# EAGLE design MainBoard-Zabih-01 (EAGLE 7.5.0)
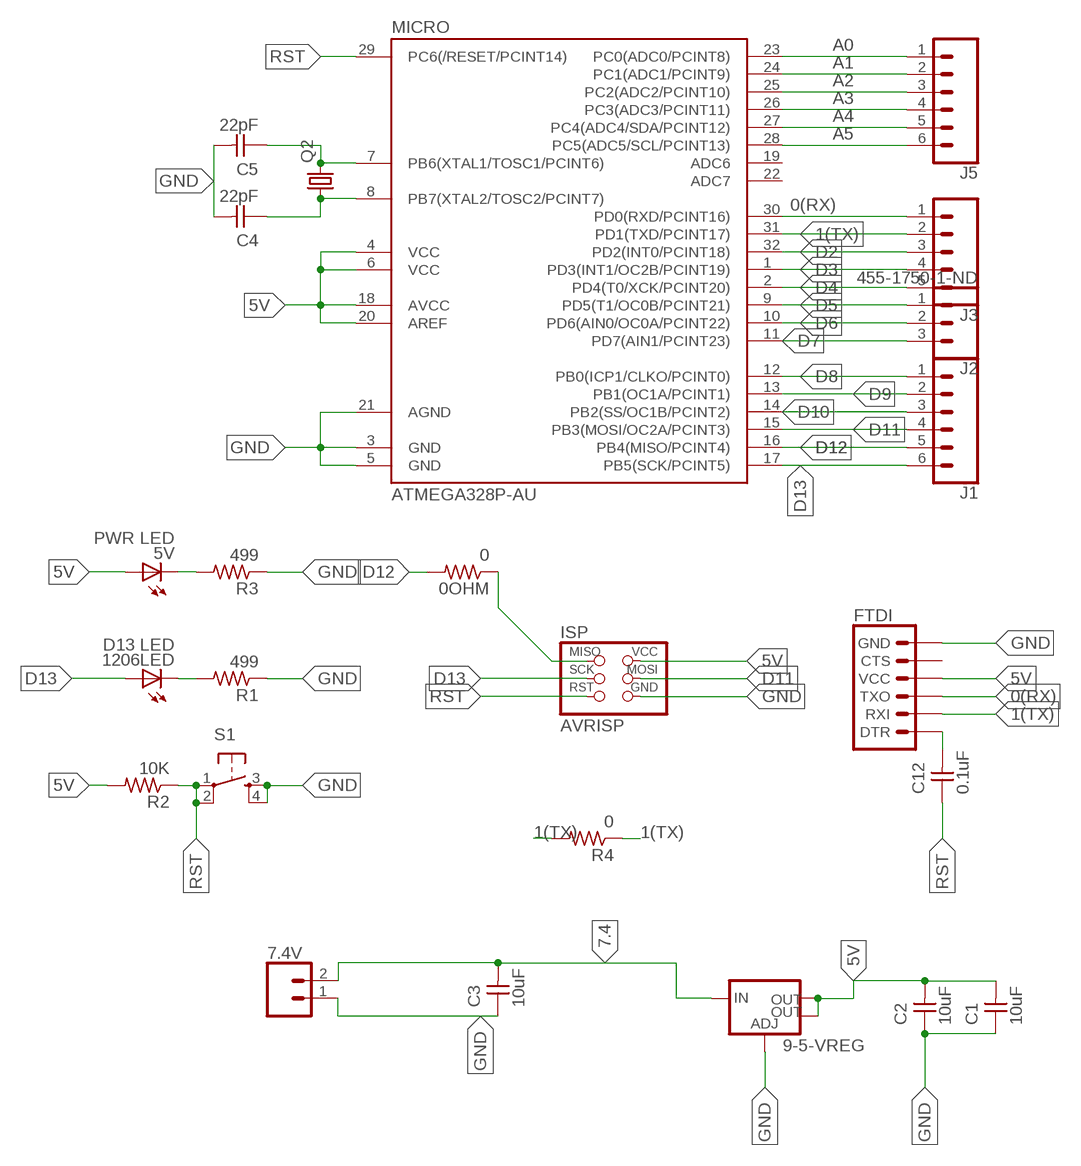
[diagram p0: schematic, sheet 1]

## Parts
0OHM  0  RES-US1206FAB  [R1206FAB]
5V  PWR LED  LEDFAB1206  [LED1206FAB]
7.4V  CONN_02LOCK  [1X02_LOCK]
9-5-VREG  V_REG_LM1117SOT223  [SOT223]
1206LED  D13 LED  LEDFAB1206  [LED1206FAB]
C1  10uF  CAP-UNPOLARIZEDFAB  [C1206FAB]
C2  10uF  CAP-UNPOLARIZEDFAB  [C1206FAB]
C3  10uF  CAP-UNPOLARIZEDFAB  [C1206FAB]
C4  22pF  CAP-UNPOLARIZEDFAB  [C1206FAB]
C5  22pF  CAP-UNPOLARIZEDFAB  [C1206FAB]
C12  0.1uF  CAP-UNPOLARIZEDFAB  [C1206FAB]
FTDI  6_PIN_SERIAL_TARGET_SILK  [1X06]
ISP  AVRISP  [2X03]
J1  CONN_06SILK_FEMALE_PTH  [1X06]
J2  455-1750-1-ND  CONN_03  [1X03]
J3  CONN_05  [1X05]
J5  CONN_06SILK_FEMALE_PTH  [1X06]
MICRO  ATMEGA328P-AU  ATMEGA48/88/168-AU  [TQFP32-08]
Q2  CRYSTALHC49U70  [HC49U70]
R1  499  RES-US1206FAB  [R1206FAB]
R2  10K  RES-US1206FAB  [R1206FAB]
R3  499  RES-US1206FAB  [R1206FAB]
R4  0  RES-US1206FAB  [R1206FAB]
S1  6MM_SWITCH6MM_SWITCH  [6MM_SWITCH]

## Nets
0(RX): FTDI.3(TXO) J3.1 MICRO.30(PD0(RXD/PCINT16))
1(TX): FTDI.2(RXI) J3.2 MICRO.31(PD1(TXD/PCINT17)) R4.1 R4.2
5V: 5V.1(A) 9-5-VREG.2(OUT) 9-5-VREG.4(OUT) C1.2 C2.2 FTDI.4(VCC) ISP.2(VCC) MICRO.4(VCC) MICRO.6(VCC) MICRO.18(AVCC) MICRO.20(AREF) R2.2
7.4: 7.4V.2 9-5-VREG.3(IN) C3.2
A0: J5.1 MICRO.23(PC0(ADC0/PCINT8))
A1: J5.2 MICRO.24(PC1(ADC1/PCINT9))
A2: J5.3 MICRO.25(PC2(ADC2/PCINT10))
A3: J5.4 MICRO.26(PC3(ADC3/PCINT11))
A4: J5.5 MICRO.27(PC4(ADC4/SDA/PCINT12))
A5: J5.6 MICRO.28(PC5(ADC5/SCL/PCINT13))
D2: J3.3 MICRO.32(PD2(INT0/PCINT18))
D3: J3.4 MICRO.1(PD3(INT1/OC2B/PCINT19))
D4: J3.5 MICRO.2(PD4(T0/XCK/PCINT20))
D5: J2.1 MICRO.9(PD5(T1/OC0B/PCINT21))
D6: J2.2 MICRO.10(PD6(AIN0/OC0A/PCINT22))
D7: J2.3 MICRO.11(PD7(AIN1/PCINT23))
D8: J1.1 MICRO.12(PB0(ICP1/CLKO/PCINT0))
D9: J1.2 MICRO.13(PB1(OC1A/PCINT1))
D10: J1.3 MICRO.14(PB2(SS/OC1B/PCINT2))
D11: ISP.4(MOSI) J1.4 MICRO.15(PB3(MOSI/OC2A/PCINT3))
D12: 0OHM.2 J1.5 MICRO.16(PB4(MISO/PCINT4))
D13: 1206LED.1(A) ISP.3(SCK) J1.6 MICRO.17(PB5(SCK/PCINT5))
GND: 7.4V.1 9-5-VREG.1(ADJ) C1.1 C2.1 C3.1 C4.2 C5.2 FTDI.6(GND) ISP.6(GND) MICRO.3(GND) MICRO.5(GND) MICRO.21(AGND) R1.1 R3.1 S1.3(S) S1.4(S1)
N$1: 1206LED.2(C) R1.2
N$2: 5V.2(C) R3.2
N$3: C5.1 MICRO.7(PB6(XTAL1/TOSC1/PCINT6)) Q2.2
N$4: C4.1 MICRO.8(PB7(XTAL2/TOSC2/PCINT7)) Q2.1
N$5: 0OHM.1 ISP.1(MISO)
N$16: C12.2 FTDI.1(DTR)
RST: C12.1 ISP.5(RST) MICRO.29(PC6(/RESET/PCINT14)) R2.1 S1.1(P) S1.2(P1)
Unconnected: FTDI.5(CTS) MICRO.19(ADC6) MICRO.22(ADC7)

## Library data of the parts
0OHM R1-R4 = fab:RES-US: Resistor (US Symbol)
5V 1206LED = fab:LED: LED
7.4V = SparkFun-Connectors:CONN_02: Multi connection point. Often used as Generic Header-pin footprint for 0.1 inch spaced/style header connections
9-5-VREG = fab:V_REG_LM1117: Voltage Regulator LM1117 Standard adjustable voltage regulator but in SMD form. Spark Fun Electronics SKU : COM-00595; PROD_ID: VREG-08170
C1-C5 C12 = fab:CAP-UNPOLARIZED
FTDI = SparkFun-Connectors:6_PIN_SERIAL_TARGET: 6-pin header connection for use with the "FTDI BASIC" pinout - TARGET SIDE. Also known as "Arduino Serial Program Header". It is used to mate with our FTDI Basic serial programmers using the Arduino IDE. Note, this device has "TARGET" in the name. It is intended to be used on a design that contains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
ISP = fab:AVRISP
J1 J5 = SparkFun-Connectors:CONN_06: Multi connection point. Often used as Generic Header-pin footprint for 0.1 inch spaced/style header connections On any of the 0.1 inch spaced packages, you can populate with these: Break Away Headers - Straight (PRT-00116) Break Away Male Headers - Right Angle (PRT-00553) Female Headers (PRT-00115)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; PROD_ID: CONN-08437
J2 = SparkFun-Connectors:CONN_03: Multi connection point. Often used as Generic Header-pin footprint for 0.1 inch spaced/style header connections On any of the 0.1 inch spaced packages, you can populate with these: Break Away Headers - Straight (PRT-00116) Break Away Male Headers - Right Angle (PRT-00553) Female Headers (PRT-00115)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; PROD_ID: XXX-00000
J3 = SparkFun-Connectors:CONN_05: Multi connection point. Often used as Generic Header-pin footprint for 0.1 inch spaced/style header connections On any of the 0.1 inch spaced packages, you can populate with these: Break Away Headers - Straight (PRT-00116) Break Away Male Headers - Right Angle (PRT-00553) Female Headers (PRT-00115)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
MICRO = atmega8:ATMEGA48/88/168
Q2 = crystal:CRYSTAL: CRYSTAL; OC_FARNELL: unknown; OC_NEWARK: unknown
S1 = fab:6MM_SWITCH: OMRON SWITCH

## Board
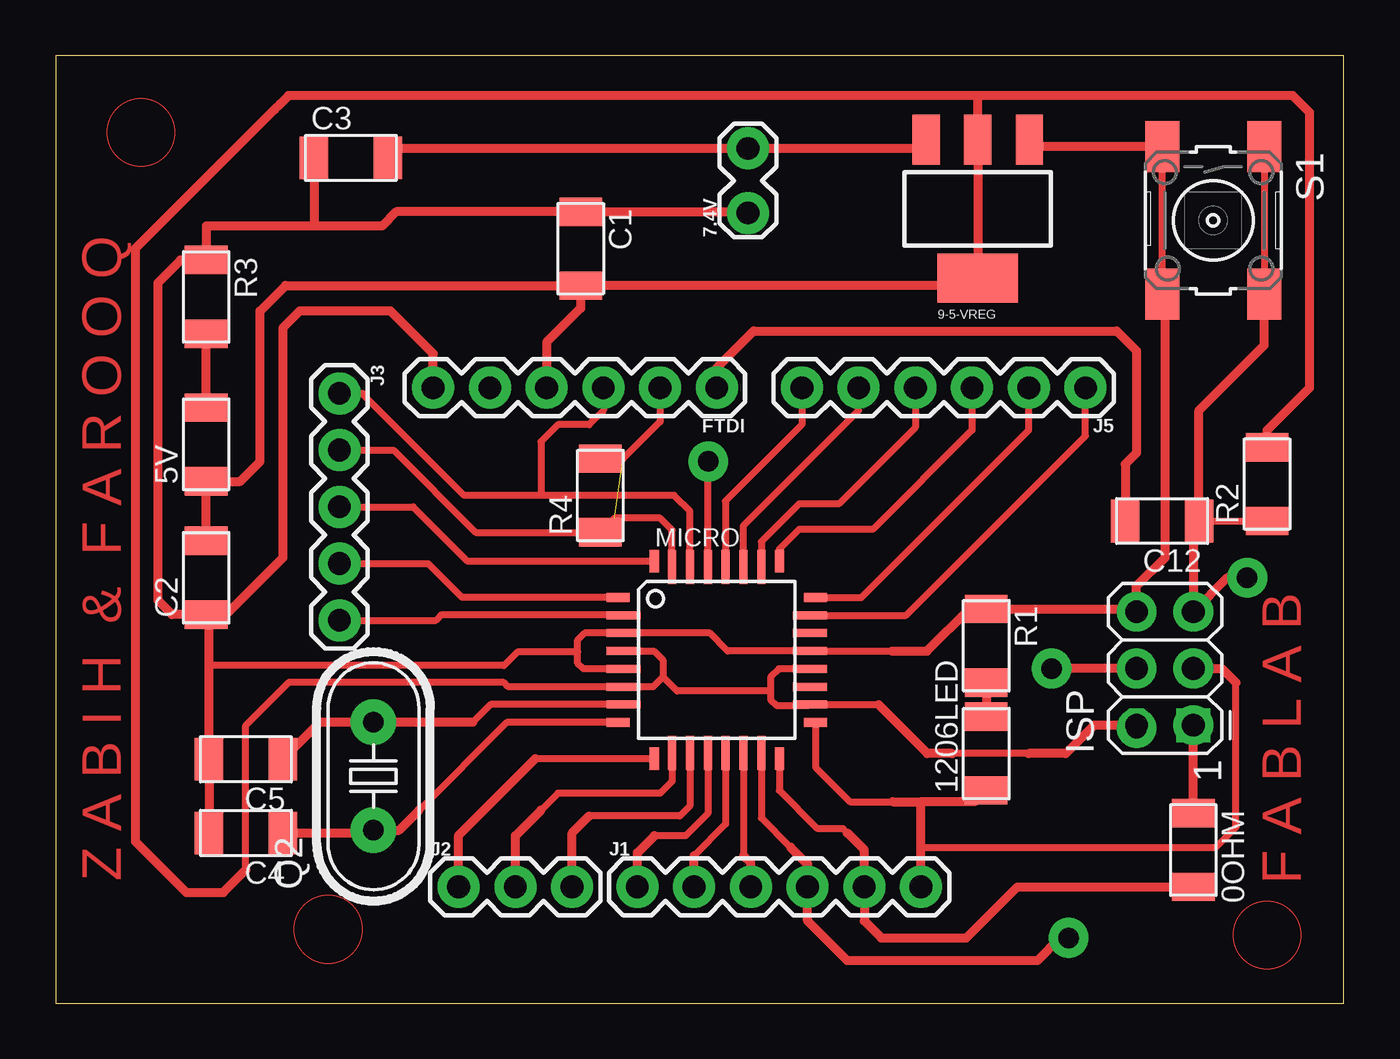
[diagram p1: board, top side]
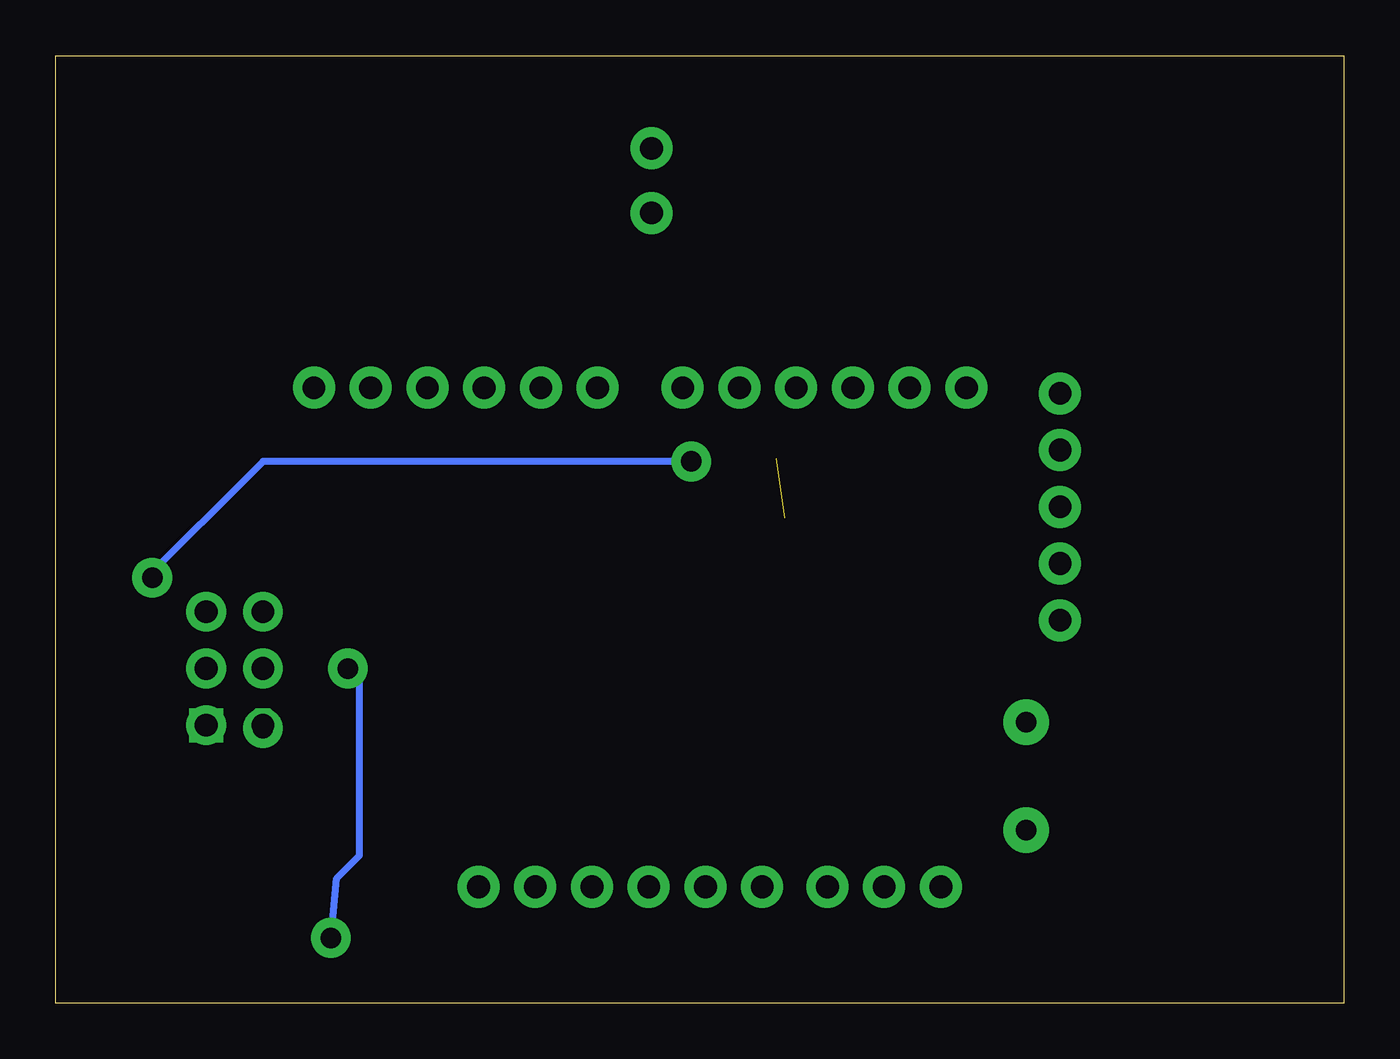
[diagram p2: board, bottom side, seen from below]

Size 57.66 x 42.42 mm. Coordinates in mm from the lower left corner, seen from the top.
Outline: 0,0 57.66,0 57.66,42.42 0,42.42 0,0
Copper layers (1*16): Top 0.035mm / dielectric 1.5mm / Bottom 0.035mm
Design rules "default *": minimum track width 10mil, minimum drill 24mil, track to track 4mil, track to pad 8mil, pad to pad 8mil, via to via 8mil, smd to smd 8mil, copper to edge 40mil, drill to drill 8mil, minimum pad ring 10mil, minimum via ring 8mil, stop-mask expansion 4mil, vias tented up to drill 0mil, thermal gap 10mil

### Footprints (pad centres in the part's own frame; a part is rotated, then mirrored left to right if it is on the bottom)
R1206FAB = smd 1.27 x 1.905: 1 -1.651,0; 2 1.651,0
LED1206FAB = smd 1.27 x 1.905: 1 -1.651,0; 2 1.651,0
1X02_LOCK = drill 1.016 pad 1.88: 1 -0.178,0; 2 2.718,0
SOT223 = smd 1.219 x 2.235: 1 -2.311,-3.099; 2 0,-3.099; 3 2.311,-3.099 | smd 3.6 x 2.2: 4 0,3.099
C1206FAB = smd 1.27 x 1.905: 1 -1.651,0; 2 1.651,0
1X06 = drill 1.016 pad 1.88: 1 0,0; 2 2.54,0; 3 5.08,0; 4 7.62,0; 5 10.16,0; 6 12.7,0
2X03 = drill 1.016 square: 1 -2.54,-1.27 | drill 1.016 octagon: 2 -2.54,1.27; 3 0,-1.27; 4 0,1.27; 5 2.54,-1.27; 6 2.54,1.27
1X03 = drill 1.016 pad 1.88: 1 0,0; 2 2.54,0; 3 5.08,0
1X05 = drill 1.016 pad 1.88: 1 0,0; 2 2.54,0; 3 5.08,0; 4 7.62,0; 5 10.16,0
TQFP32-08 = smd 1.016 x 0.406: 1 -4.42,2.8; 8 -4.42,-2.8; 17 4.42,-2.8; 24 4.42,2.8 | smd 1.524 x 0.356: 2 -4.166,2; 3 -4.166,1.2; 4 -4.166,0.4; 5 -4.166,-0.4; 6 -4.166,-1.2; 7 -4.166,-2; 18 4.166,-2; 19 4.166,-1.2; 20 4.166,-0.4; 21 4.166,0.4; 22 4.166,1.2; 23 4.166,2 | smd 0.406 x 1.016: 9 -2.8,-4.42; 16 2.8,-4.42; 25 2.8,4.42; 32 -2.8,4.42 | smd 0.356 x 1.524: 10 -2,-4.166; 11 -1.2,-4.166; 12 -0.4,-4.166; 13 0.4,-4.166; 14 1.2,-4.166; 15 2,-4.166; 26 2,4.166; 27 1.2,4.166; 28 0.4,4.166; 29 -0.4,4.166; 30 -1.2,4.166; 31 -2,4.166
HC49U70 = drill 0.813: 1 -2.413,0; 2 2.413,0
6MM_SWITCH = smd 2.286 x 1.524: 1 -3.302,2.286; 2 3.302,2.286; 3 -3.302,-2.286; 4 3.302,-2.286

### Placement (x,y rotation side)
0OHM  50.93,6.86 270 top
5V  6.73,25.02 90 top
7.4V  30.99,35.56 90 top
9-5-VREG  41.27,35.56 180 top
1206LED  41.66,11.18 90 top
C1  23.5,33.78 270 top
C2  6.73,19.05 90 top
C3  13.21,37.85 0 top
C4  8.51,7.62 180 top
C5  8.51,10.92 180 top
C12  49.53,21.59 180 top
FTDI  29.59,27.56 180 top
ISP  49.66,14.99 90 top
J1  26.04,5.21 0 top
J2  18.03,5.21 0 top
J3  12.7,27.3 270 top
J5  46.1,27.56 180 top
MICRO  29.59,15.37 0 top
Q2  14.22,10.16 90 top
R1  41.66,16 270 top
R2  54.23,23.24 90 top
R3  6.73,31.62 270 top
R4  24.38,22.73 90 top
S1  51.82,35.05 270 top

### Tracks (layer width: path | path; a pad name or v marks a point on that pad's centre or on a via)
0(RX)
  Top 0.305: MICRO.30 28.39,22.03 27.69,22.73 21.72,22.73 | 21.72,22.73 18.29,22.73 13.72,27.3 J3.1 | FTDI.3 24.51,26.54 23.88,25.91 22.48,25.91 21.72,25.15 21.72,22.73
1(TX)  (1 unrouted)
  Top 0.305: FTDI.2 27.05,26.04 25.4,24.38 R4.2 | MICRO.31 27.59,21.18 27.05,21.72 25.02,21.72 R4.1 18.8,21.08 15.11,24.77 J3.2
5V
  Top 0.305: 33.74,14.99 MICRO.20 32.37,14.97 32,14.61 32,13.97 | 25.44,15.75 MICRO.4 26.78,15.77 27.18,15.37 27.18,14.61 | 32,13.97 32,13.59 32.26,13.34 33.73,13.34 MICRO.18 36.83,13.37 | 27.18,14.61 26.74,14.17 MICRO.6 20.25,14.17 20.07,14.35 10.41,14.35 8.51,12.45 8.51,5.97 | 32,13.97 27.81,13.97 27.18,14.61 | 43.56,11.18 40.13,11.18
  Top 0.406: C1.2 10.29,32.13 9.14,30.99 9.14,24.26 8.26,23.37 5V.1 C2.2 | C1.2 23.5,31.11 21.97,29.59 FTDI.4 | C1.2 41.22,32.13 9-5-VREG.4 9-5-VREG.2 41.27,40.64 | R2.2 54.23,25.65 56.13,27.56 56.13,39.88 55.37,40.64 41.27,40.64 | 8.51,5.97 7.49,4.95 5.84,4.95 3.56,7.24 3.56,33.78 9.78,40.01 10.03,40.26 10.41,40.64 41.27,40.64 | ISP.2 46.48,12.45 45.21,11.18 43.56,11.18 | 40.13,11.18 39.02,11.18 36.83,13.37
7.4
  Top 0.406: 14.73,37.72 C3.2 15.29,38.28 7.4V.2 38.58,38.28 9-5-VREG.3
A0
  Top 0.305: MICRO.23 38.07,17.37 46.1,25.4 J5.1
A1
  Top 0.305: MICRO.24 36.07,18.16 43.56,25.65 J5.2
A2
  Top 0.305: MICRO.25 32.39,20.33 33.27,21.21 36.58,21.21 41.02,25.65 J5.3
A3
  Top 0.305: J5.4 38.48,25.78 35.05,22.35 33.27,22.35 31.59,20.67 MICRO.26
A4
  Top 0.305: 35.94,27.18 J5.5 35.94,26.54 30.79,21.39 MICRO.27
A5
  Top 0.305: J5.6 33.4,25.91 29.97,22.48 29.97,19.55 MICRO.28
D2
  Top 0.305: MICRO.32 18.44,19.79 16,22.23 J3.3
D3
  Top 0.305: MICRO.1 18.19,18.17 16.67,19.68 J3.4
D4
  Top 0.305: MICRO.2 25.39,17.4 17.27,17.4 17.02,17.14 J3.5
D5
  Top 0.305: MICRO.9 21.46,10.95
  Top 0.406: J2.1 18.03,7.52 21.46,10.95
D6
  Top 0.305: MICRO.10 27.59,9.94 27.05,9.4 22.48,9.4 21.72,8.64
  Top 0.406: J2.2 20.57,7.49 21.72,8.64
D7
  Top 0.305: MICRO.11 28.39,8.83 27.94,8.38 23.88,8.38
  Top 0.406: J2.3 23.11,7.62 23.88,8.38
D8
  Top 0.305: MICRO.12 29.19,8.49 28.19,7.49 26.8,7.49
  Top 0.406: J1.1 26.04,6.73 26.8,7.49
D9
  Top 0.305: 28.57,6.6 29.99,8.02 MICRO.13
  Top 0.406: J1.2 28.57,6.6
D10
  Top 0.305: MICRO.14 30.79,6.6
  Top 0.406: J1.3 31.11,6.28 30.79,6.6
D11  (via drill 0.91 pad 1.78)
  Top 0.305: MICRO.15 31.59,8.29 32.89,6.99
  Top 0.406: 32.89,6.99 33.66,6.22 J1.4 33.66,3.68 35.43,1.91 43.94,1.91 44.96,2.92 v45.34,2.92 | ISP.4 v44.58,14.99
  Bottom 0.305: v45.34,2.92 45.09,5.59 44.07,6.6 44.07,14.48 v44.58,14.99
D12
  Top 0.305: MICRO.16 32.39,9.52 34.1,7.81 35.24,7.81 35.43,7.62
  Top 0.406: 35.43,7.62 36.2,6.86 J1.5 36.2,3.68 36.96,2.92 40.77,2.92 43.05,5.21 0OHM.2
D13
  Top 0.305: MICRO.17 34.01,10.57 35.56,9.02 37.47,9.02 37.72,9.02 | 38.73,6.99 51.94,6.99 52.83,7.87 52.83,14.35
  Top 0.406: 41.15,9.53 1206LED.1 41.15,9.02 38.73,9.02 | 37.47,9.02 38.73,9.02 | J1.6 38.73,6.99 38.73,9.02 | ISP.3 52.2,14.99 52.83,14.35
GND
  Top 0.305: 37.45,15.77 MICRO.21 30.08,15.77 29.28,16.57 MICRO.3 23.68,16.57 23.37,16.26 23.37,15.75 | S1.4 S1.3 | MICRO.5 23.62,14.97 23.37,15.22 23.37,15.75 | 6.86,15.11 20.07,15.11 20.7,15.75 23.37,15.75
  Top 0.406: 11.56,37.08 C3.1 11.56,34.92 11.43,34.8 | S1.4 49.66,31.62 49.66,19.94 48.39,18.67 ISP.6 48.26,17.65 R1.1 40.89,17.65 39.01,15.77 37.45,15.77 | C2.1 6.1,17.4 | 11.43,34.8 14.61,34.8 15.24,35.43 C1.1 30.94,35.43 7.4V.1 | 11.43,34.8 6.73,34.8 R3.1 5.59,33.27 4.57,32.26 4.57,18.03 5.21,17.4 C2.1 | S1.3 43.66,38.35 9-5-VREG.1 | 6.86,17.27 6.86,15.11 C5.2 C4.2 | 6.86,17.27 C2.1 | FTDI.6 16.89,29.08 14.99,30.99 10.92,30.99 10.16,30.23 10.16,19.94 7.49,17.27 6.86,17.27
N$1
  Top 0.406: R1.2 1206LED.2
N$2
  Top 0.406: 5V.2 R3.2
N$3
  Top 0.305: MICRO.7 19.46,13.37 18.67,12.57
  Top 0.406: 10.41,10.67 C5.1 11.81,12.57 Q2.2 18.67,12.57
N$4
  Top 0.305: MICRO.8 20.19,12.57 16.26,8.64
  Top 0.406: C4.1 14.1,7.62 Q2.1 15.37,7.75 16.26,8.64
N$5
  Top 0.406: 0OHM.1 ISP.1
N$6  (via drill 0.91 pad 1.78)
  other vias: 48.39,17.53
N$7  (via drill 0.91 pad 1.78)
  other vias: 48.39,14.99
N$8  (via drill 0.91 pad 1.78)
  other vias: 50.93,14.99
N$9  (via drill 0.91 pad 1.78)
  other vias: 50.93,12.45
N$10  (via drill 0.91 pad 1.78)
  other vias: 48.39,12.32
N$11  (via drill 0.91 pad 2.03)
  other vias: 14.22,7.75
N$12  (via drill 0.91 pad 2.03)
  other vias: 14.22,12.57
N$16
  Top 0.406: C12.2 47.88,24.13 48.39,24.64 48.39,29.21 47.5,30.1 31.24,30.1 29.59,28.45 FTDI.1
RST  (via drill 0.91 pad 1.78)
  Top 0.305: S1.2 54.1,31.88 S1.1 54.61,37.85 | 29.21,19.55 MICRO.29 29.19,24.24 v29.21,24.26 | C12.1 R2.1
  Top 0.406: 54.1,31.88 54.1,29.46 51.18,26.54 C12.1 50.93,21.34 ISP.5 52.45,19.05 v53.34,19.05
  Bottom 0.305: v29.21,24.26 48.39,24.26 53.98,18.67 v53.34,19.05
  other vias: 50.93,17.53
(copper drawn outside any net)
  shapes: Top circle x3

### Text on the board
Top: Z A B I H & F A R O O Q | F A B L A B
